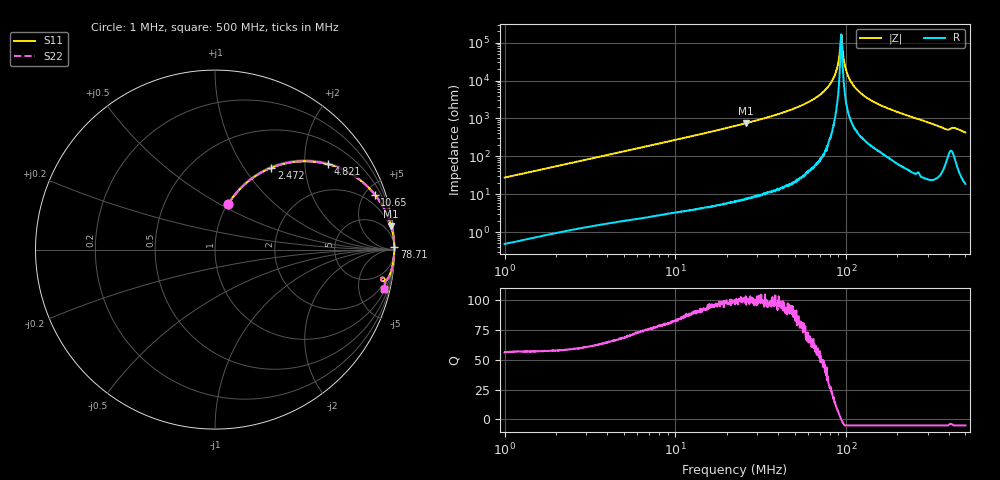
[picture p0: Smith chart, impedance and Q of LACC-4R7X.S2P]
!s-Parameter Generated by FASTRON Sdn. Bhd.
!FASTRON P/N : LACC-4R7X
!Keysight Technologies,E4991B,MY54100416,A.01.15
!Date: Wed Mar 18 09:13:22 2026
!Version  : Rev00 Wed Mar 18 09:13:22 2026
!Data & Calibration Information:
!PortZ  Port1:50+j0  Port2:50+j0
!When reading, reference impedance value at option line is always used.
!Remarks : This data is being provided solely for informational purposes.
!Freq	S11	S21	S12	S22
# Hz S dB R 50
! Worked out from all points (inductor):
!   1601 points, 1 MHz to 500 MHz, reference 50 ohm
!   read as one part in series: L = 4.35 uH near 1.032 MHz
!   highest Q = 101 at 25.82 MHz (marker M1), where L = 4.58 uH
!   self-resonance near 93.74 MHz
!   S11 on the Smith chart (normalised r, x): 1 MHz: 1.01, +0.55; 2.472 MHz: 1.02, +1.34; 4.821 MHz: 1.04, +2.60; 10.65 MHz: 1.07, +5.77; 78.71 MHz: open; 500 MHz: 1.37, -8.52
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1000000  -11.60 73.7  -0.35 -15.2  -0.35 -15.2  -11.60 73.7
2471938  -5.15 55.5  -1.68 -33.6  -1.68 -33.6  -5.15 55.5
2820919  -4.40 52.0  -2.07 -37.1  -2.07 -37.1  -4.40 52.0
4821440  -2.08 37.2  -4.37 -51.9  -4.37 -51.9  -2.08 37.2
7957584  -0.89 24.8  -7.54 -64.5  -7.54 -64.5  -0.89 24.8
1.064867e7  -0.52 19.0  -9.73 -70.3  -9.73 -70.3  -0.52 19.0
2.236068e7  -0.12 9.0  -16.12 -80.4  -16.12 -80.4  -0.12 9.0
2.581658e7  -0.09 7.7  -17.51 -81.8  -17.51 -81.8  -0.09 7.7
6.307767e7  -0.01 1.9  -29.62 -87.2  -29.62 -87.2  -0.01 1.9
7.870937e7  -0.00 0.8  -36.81 -87.4  -36.81 -87.4  -0.00 0.8
8.673569e7  -0.00 0.4  -43.77 -85.0  -43.77 -85.0  -0.00 0.4
8.912629e7  -0.00 0.2  -47.47 -82.3  -47.47 -82.3  -0.00 0.2
9.193919e7  -0.01 0.1  -55.26 -69.4  -55.26 -69.4  -0.01 0.1
9.374216e7  -0.01 0.0  -64.30 -4.2  -64.30 -4.2  -0.01 0.0
9.558049e7  -0.01 -0.1  -55.41 68.5  -55.41 68.5  -0.01 -0.1
9.859709e7  -0.01 -0.2  -47.60 79.5  -47.60 79.5  -0.01 -0.2
1.013146e8  -0.01 -0.4  -43.89 82.3  -43.89 82.3  -0.01 -0.4
1.116461e8  -0.01 -0.8  -36.88 84.5  -36.88 84.5  -0.01 -0.8
1.33487e8  -0.02 -1.7  -30.69 84.6  -30.69 84.6  -0.02 -1.7
1.77937e8  -0.04 -3.2  -25.15 84.0  -25.15 84.0  -0.04 -3.2
3.794925e8  -0.32 -10.4  -14.79 73.4  -14.79 73.4  -0.32 -10.4
5e8  -0.32 -13.1  -12.92 74.4  -12.92 74.4  -0.32 -13.1
